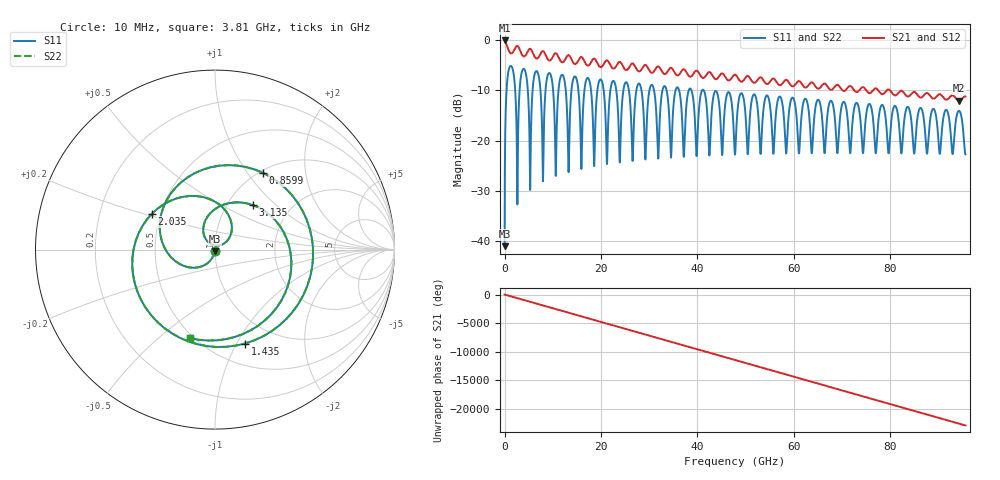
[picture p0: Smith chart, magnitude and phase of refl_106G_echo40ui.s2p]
! Created with skrf 1.10.0 (http://scikit-rf.org).
# GHz S RI R 50.0
!freq ReS11 ImS11 ReS21 ImS21 ReS12 ImS12 ReS22 ImS22
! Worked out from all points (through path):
!   3826 points, 10 MHz to 95.62 GHz, reference 50 ohm
!   highest |S21| = -0.06 dB at 10 MHz (marker M1); lowest = -12.1 dB at 94.33 GHz (marker M2)
!   group delay of S21, straight-line fit = 666 ps
!   lowest |S11| = -41.0 dB at 10 MHz (marker M3), VSWR 1.02, Z = 49.8 - j0.87 ohm
!   |S11| at or under -10 dB: 36.22 GHz to 38.22 GHz (1.997 GHz wide, 5.37 % of centre); 38.8 GHz to 40.99 GHz (2.19 GHz wide, 5.49 % of centre); 41.34 GHz to end of sweep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
!   |S22| runs from -41.0 to -5.1 dB; largest |S21 - S12| = 3.7e-16
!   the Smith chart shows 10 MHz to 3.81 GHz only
!   S11 on the Smith chart (normalised r, x): 10 MHz: 1.00, -0.02; 859.9 MHz: 1.03, +1.19; 1.435 GHz: 0.72, -1.08; 2.035 GHz: 0.45, +0.21; 3.135 GHz: 1.30, +0.72; 3.81 GHz: 0.48, -0.64
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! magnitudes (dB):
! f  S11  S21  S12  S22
! 10 MHz  -41.0  -0.1  -0.1  -41.0
! 859.9 MHz  -5.9  -2.0  -2.0  -5.9
! 1.435 GHz  -5.2  -2.6  -2.6  -5.2
! 2.035 GHz  -7.9  -1.9  -1.9  -7.9
! 3.135 GHz  -9.8  -1.9  -1.9  -9.8
! 3.81 GHz  -5.8  -3.1  -3.1  -5.8
! 5.284 GHz  -28.4  -1.7  -1.7  -28.4
! 6.634 GHz  -6.2  -3.7  -3.7  -6.2
! 7.934 GHz  -26.8  -2.2  -2.2  -26.8
! 9.284 GHz  -6.5  -4.1  -4.1  -6.5
! 15.96 GHz  -25.4  -3.3  -3.3  -25.4
! 17.26 GHz  -7.5  -5.1  -5.1  -7.5
! 18.58 GHz  -25.1  -3.7  -3.7  -25.1
! 19.91 GHz  -7.8  -5.4  -5.4  -7.8
! 21.23 GHz  -24.6  -4.0  -4.0  -24.6
! 31.88 GHz  -23.6  -5.2  -5.2  -23.6
! 33.21 GHz  -9.1  -6.8  -6.8  -9.1
! 47.83 GHz  -22.7  -6.9  -6.9  -22.7
! 63.75 GHz  -22.5  -8.4  -8.4  -22.5
! 79.7 GHz  -22.5  -9.8  -9.8  -22.5
! 94.33 GHz  -14.1  -12.1  -12.1  -14.1
! 95.62 GHz  -22.7  -11.2  -11.2  -22.7
